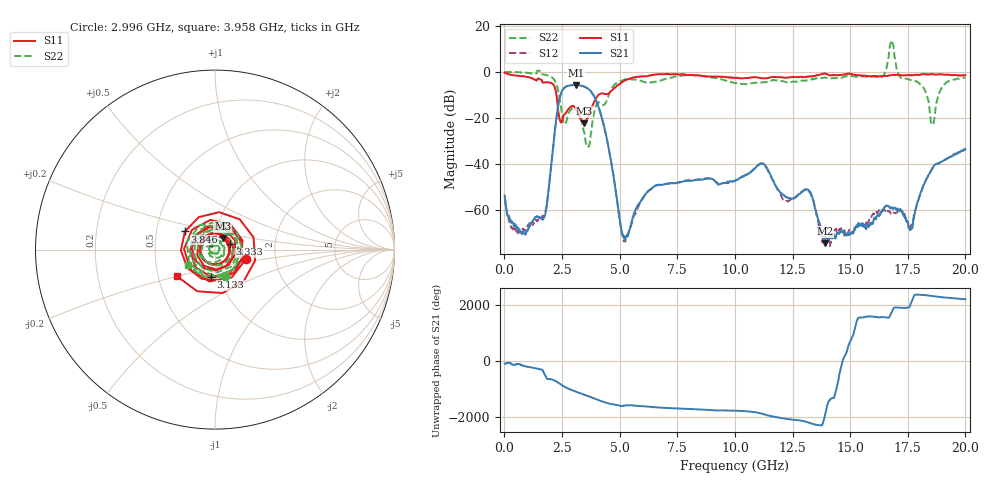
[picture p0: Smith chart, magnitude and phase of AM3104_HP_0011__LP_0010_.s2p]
!Created with skrf (http://scikit-rf.org).
# Hz S RI R 50.0
!freq ReS11 ImS11 ReS21 ImS21 ReS12 ImS12 ReS22 ImS22
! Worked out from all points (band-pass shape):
!   1601 points, 10 MHz to 20 GHz, reference 50 ohm
!   highest |S21| = -5.62 dB at 3.108 GHz (marker M1); lowest = -74.5 dB at 13.92 GHz (marker M2)
!   |S21| within 3 dB of the highest: 2.483 GHz to 3.768 GHz (1.284 GHz wide, 41.1 % of centre)
!   lowest |S11| = -22.3 dB at 3.458 GHz (marker M3), VSWR 1.17, Z = 54 + j6.91 ohm
!   |S11| at or under -10 dB: 2.259 GHz to 4.08 GHz (1.821 GHz wide, 57.4 % of centre)
!   |S22| runs from -32.7 to 13.7 dB; largest |S21 - S12| = 0.029
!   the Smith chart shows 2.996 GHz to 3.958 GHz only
!   S11 on the Smith chart (normalised r, x): 2.996 GHz: 1.40, -0.16; 3.133 GHz: 0.91, -0.28; 3.333 GHz: 1.18, +0.07; 3.846 GHz: 0.70, +0.15; 3.958 GHz: 0.63, -0.20
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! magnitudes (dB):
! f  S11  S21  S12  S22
! 10 MHz  -0.4  -53.6  -54.8  -0.1
! 759.6 MHz  -1.8  -70.5  -68.3  -0.3
! 1.697 GHz  -4.6  -63.7  -62.4  -1.1
! 2.396 GHz  -20.5  -11.4  -11.4  -11.3
! 2.996 GHz  -14.9  -5.7  -5.7  -15.9
! 3.108 GHz  -16.0  -5.6  -5.6  -16.6
! 3.133 GHz  -16.3  -5.7  -5.6  -16.9
! 3.333 GHz  -21.1  -5.9  -6.0  -20.4
! 3.346 GHz  -21.4  -5.9  -6.0  -20.9
! 3.458 GHz  -22.3  -6.3  -6.3  -25.9
! 3.846 GHz  -14.2  -9.7  -9.7  -20.0
! 3.958 GHz  -11.7  -12.0  -12.0  -15.2
! 5.17 GHz  -4.0  -71.0  -73.5  -3.5
! 6.682 GHz  -1.0  -49.0  -49.1  -4.0
! 10.01 GHz  -2.6  -47.3  -47.4  -4.8
! 11.19 GHz  -2.8  -39.8  -39.9  -4.5
! 13.34 GHz  -2.0  -53.8  -54.0  -3.3
! 13.92 GHz  -0.6  -74.5  -71.4  -2.4
! 16.68 GHz  -1.6  -58.5  -60.6  7.2
! 17.63 GHz  -1.4  -68.0  -67.5  -3.5
! 18.58 GHz  -0.9  -41.7  -41.8  -22.9
! 20 GHz  -1.4  -33.7  -33.3  -2.5
